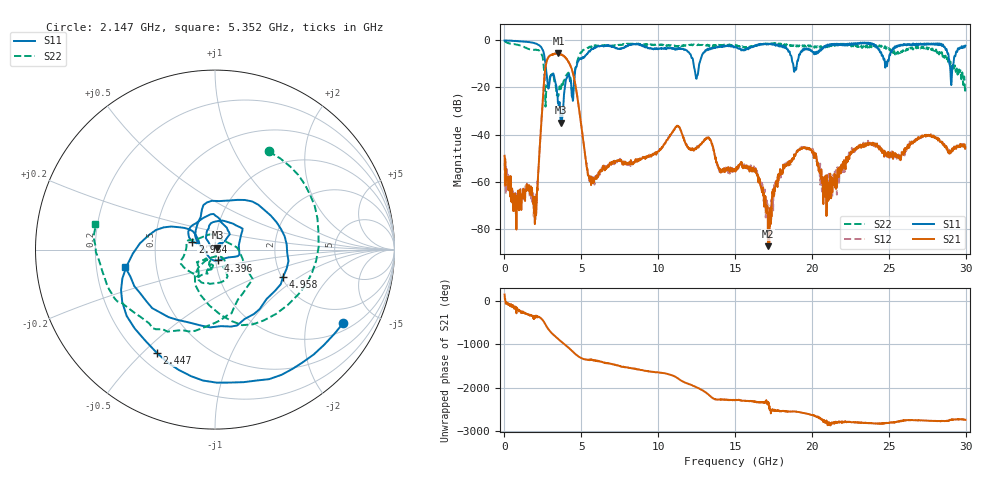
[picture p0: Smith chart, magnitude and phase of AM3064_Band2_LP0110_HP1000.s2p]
# Hz S DB R 50.0
!freq dBS11 angS11 dBS21 angS21 dBS12 angS12 dBS22 angS22
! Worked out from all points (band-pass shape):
!   1600 points, 10 MHz to 29.98 GHz, reference 50 ohm
!   highest |S21| = -5.57 dB at 3.515 GHz (marker M1); lowest = -87.3 dB at 17.14 GHz (marker M2)
!   |S21| within 3 dB of the highest: 2.762 GHz to 4.118 GHz (1.356 GHz wide, 39.4 % of centre)
!   lowest |S11| = -34.9 dB at 3.684 GHz (marker M3), VSWR 1.04, Z = 51.4 + j1.2 ohm
!   |S11| at or under -10 dB: 2.669 GHz to 4.727 GHz (2.058 GHz wide, 55.7 % of centre); 12.3 GHz to 12.67 GHz (372.7 MHz wide, 2.98 % of centre); 28.95 GHz to 29.2 GHz (256.3 MHz wide, 0.882 % of centre)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
!   |S22| runs from -28.1 to -0.2 dB; largest |S21 - S12| = 0.013
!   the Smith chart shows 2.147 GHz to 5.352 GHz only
!   S11 on the Smith chart (normalised r, x): 2.147 GHz: 1.30, -3.30; 2.447 GHz: 0.27, -0.55; 2.934 GHz: 0.77, +0.07; 4.396 GHz: 1.03, -0.12; 4.958 GHz: 2.05, -0.74; 5.352 GHz: 0.33, -0.09
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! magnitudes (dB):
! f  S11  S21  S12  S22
! 10 MHz  0.0  -49.0  -52.1  -0.2
! 684.8 MHz  -0.2  -64.9  -69.1  -1.7
! 2.147 GHz  -1.7  -63.7  -62.1  -4.1
! 2.447 GHz  -3.6  -29.4  -29.5  -6.4
! 2.934 GHz  -17.5  -6.6  -6.6  -16.3
! 3.515 GHz  -27.0  -5.6  -5.6  -23.3
! 3.684 GHz  -34.9  -6.0  -5.9  -20.1
! 4.396 GHz  -24.1  -12.7  -12.5  -21.0
! 4.958 GHz  -7.8  -34.2  -34.1  -5.2
! 5.015 GHz  -8.0  -36.9  -36.8  -5.1
! 5.352 GHz  -5.9  -53.7  -53.3  -3.3
! 10 GHz  -3.5  -47.1  -46.7  -1.9
! 11.27 GHz  -3.7  -36.2  -36.2  -2.6
! 12.47 GHz  -16.2  -45.8  -45.7  -1.9
! 15 GHz  -2.6  -55.4  -55.4  -2.0
! 16.34 GHz  -2.4  -54.5  -54.1  -2.4
! 17.14 GHz  -1.6  -87.3  -77.3  -1.4
! 19.99 GHz  -4.4  -46.8  -47.0  -2.2
! 21.1 GHz  -2.3  -60.6  -56.6  -2.5
! 23.01 GHz  -1.4  -45.8  -45.2  -2.7
! 25 GHz  -8.3  -48.6  -48.4  -3.2
! 29.98 GHz  -2.2  -45.4  -45.6  -20.3
